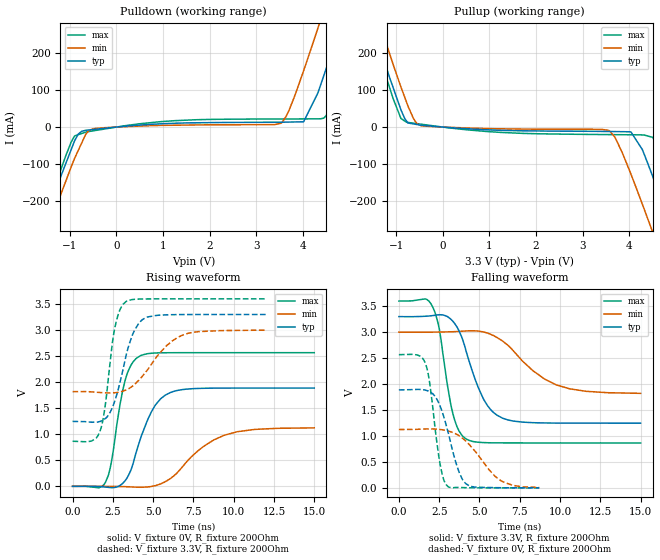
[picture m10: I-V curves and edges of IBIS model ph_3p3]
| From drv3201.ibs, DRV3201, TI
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|   ph_3p3 Model
[Model]   ph_3p3
Model_type   Output
Polarity   Non-Inverting
Vmeas = 1.65
Vref = 0
Cref = 2pF
Rref = 350
|   typ   min   max
|   (nom PVT)   (fast PVT)   (slow PVT)
 C_comp   1.346e-12   1.334e-12   1.378e-12
| Where nom  PVT is Nominal Process, 3.3V, 27C
|   Fast PVT is Strong Process,  3.6V, -40C
|   Slow PVT is Weak Process,   3V, 150C
[Voltage Range]   3.3   3   3.6
|Junction Temperature
[Temperature Range]   27   150   -40
[Pullup Reference]   3.3   3   3.6
[Pulldown Reference]   0   0   0
[Power Clamp Reference]   3.3   3   3.6
[GND Clamp Reference]   0   0   0
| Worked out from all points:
|   slope of the pulldown table from 0 to 0.495 V, typ, clamps not added: 94.8 ohm
|   slope of the pullup table from 0 to 0.495 V, typ, clamps not added: 115 ohm
|   falling waveform, V_fixture 3.3V, R_fixture 200Ohm: 20-80 % time 1.43ns typ, 2.59ns min, 853ps max; typ from 3.3 V to 1.25 V
|   rising waveform, V_fixture 0V, R_fixture 200Ohm: 20-80 % time 1.35ns typ, 2.44ns min, 844ps max; typ from 0 V to 1.89 V
|   rising waveform, V_fixture 3.3V, R_fixture 200Ohm: 20-80 % time 1.05ns typ, 1.91ns min, 668ps max; typ from 1.25 V to 3.3 V
|   falling waveform, V_fixture 0V, R_fixture 200Ohm: 20-80 % time 1.01ns typ, 1.79ns min, 630ps max; typ from 1.89 V to 0 V
[Pulldown]
|   Voltage   I(typ)   I(min)   I(max)
-3.3V     -923mA     -940.4mA   -934.1mA
-1.555V   -263.4mA   -307.7mA   -249.2mA
-972mV    -61.23mA   -107.8mA   -40.83mA
-745.8mV  -11.37mA   -43.12mA   -17.33mA
-477mV    -6.297mA   -3.97mA    -9.725mA
3.525V    13.06mA    10.05mA    21.79mA
4.013V    14.28mA    151.4mA    21.94mA
4.316V    90.97mA    264.9mA    22.14mA
4.446V    138.4mA    314.5mA    23.97mA
4.716V    242.4mA    418.9mA    101.4mA
5.213V    435.8mA    614.8mA    292.7mA
6.6V      989.9mA    1.162A     849.8mA
[Pullup]
|   Voltage   I(typ)   I(min)   I(max)
-3.3V     1.001A     1.052A     983.4mA
-1.574V   303.7mA    366.1mA    278.6mA
-1.415V   241.5mA    304.7mA    213.6mA
-896.4mV  46.57mA    108.3mA    23.23mA
-745.8mV  10.99mA    57mA       12.51mA
-456mV    4.901mA    3.428mA    7.633mA
3.573V    -12.03mA   -10.08mA   -20.39mA
4.036V    -13.41mA   -128mA     -20.84mA
4.496V    -132mA     -283.2mA   -27.74mA
4.694V    -202.9mA   -353mA     -81.46mA
5.178V    -376.3mA   -523.9mA   -254.2mA
6.6V      -909.4mA   -1.04A     -801.1mA
[Ramp]
R_load = 200
|   typ   min   max
dV/dt_r   1.13263/1.34178e-09   0.673529/2.42925e-09   1.53974/8.42057e-10
dV/dt_f   1.23188/1.42835e-09   0.707193/2.55651e-09   1.64047/8.52289e-10
[Falling Waveform]
V_fixture = 3.3V
V_fixture_min = 3V
V_fixture_max = 3.6V
R_fixture = 200Ohm
|   Time   V(typ)   V(min)   V(max)
0s        3.3V       3V         3.6V
1.632ns   3.307V     2.999V     3.642V
2.09ns    3.32V      3.001V     3.492V
2.506ns   3.335V     3.003V     3.066V
3.366ns   3.205V     3.009V     1.412V
4.22ns    2.582V     3.024V     934.3mV
5.3ns     1.685V     3.001V     871.8mV
6.478ns   1.338V     2.819V     866.3mV
9.764ns   1.248V     1.985V     865.9mV
15ns      1.247V     1.821V     865.9mV
[Rising Waveform]
V_fixture = 0V
V_fixture_min = 0V
V_fixture_max = 0V
R_fixture = 200Ohm
|   Time   V(typ)   V(min)   V(max)
0s        934.8pV    256.4nV    687.4pV
2.056ns   -14.65mV   524.8uV    86.62mV
2.41ns    -26.59mV   -703.4uV   467.3mV
2.96ns    19.8mV     -4.105mV   1.597V
3.26ns    107.2mV    -6.713mV   2.032V
4.178ns   880.9mV    -17.77mV   2.503V
5.174ns   1.575V     16.17mV    2.561V
6.256ns   1.821V     192.8mV    2.566V
9.404ns   1.887V     980.1mV    2.566V
15ns      1.888V     1.123V     2.566V
[Rising Waveform]
V_fixture = 3.3V
V_fixture_min = 3V
V_fixture_max = 3.6V
R_fixture = 200Ohm
|   Time   V(typ)   V(min)   V(max)
0s        1.247V     1.818V     865.9mV
1.688ns   1.244V     1.803V     1.045V
2ns       1.293V     1.796V     1.487V
2.626ns   1.642V     1.797V     3.047V
2.94ns    1.988V     1.812V     3.39V
3.348ns   2.547V     1.853V     3.556V
3.872ns   3.011V     1.963V     3.592V
4.646ns   3.252V     2.235V     3.599V
6.832ns   3.299V     2.905V     3.6V
11.98ns   3.3V       3V         3.6V
[Falling Waveform]
V_fixture = 0V
V_fixture_min = 0V
V_fixture_max = 0V
R_fixture = 200Ohm
|   Time   V(typ)   V(min)   V(max)
0s        1.888V     1.124V     2.566V
1.144ns   1.898V     1.128V     2.56V
1.644ns   1.883V     1.135V     2.402V
1.91ns    1.853V     1.136V     2.026V
2.526ns   1.601V     1.126V     513.8mV
2.996ns   1.139V     1.1V       39.79mV
3.62ns    405.4mV    1.026V     7.136mV
4.16ns    78.54mV    898.8mV    3.226mV
6.218ns   2.665mV    161mV      2.859uV
8.706ns   70.67uV    8.545mV    187.5nV
